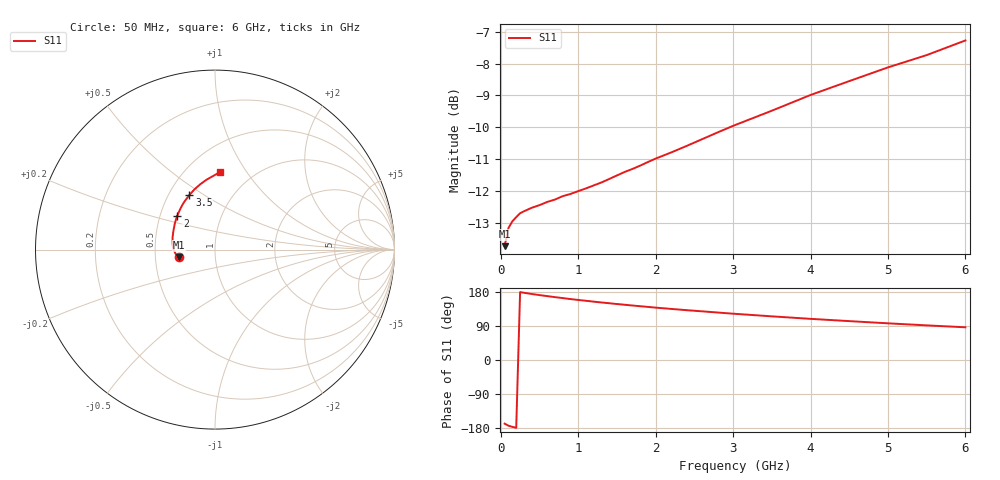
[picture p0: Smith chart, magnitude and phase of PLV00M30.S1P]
! Infineon Technologies  Discrete & RF Semiconductors
! BAR 64-04W /-05W /-06W
! Si PIN Diode in SOT323
! IF = 0.3 mA
! S-Parameters:  October  2008
# GHz  S  MA  R  50
!  f  S11
! GHz  MAG  ANG
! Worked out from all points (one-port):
!   34 points, 50 MHz to 6 GHz, reference 50 ohm
!   lowest |S11| = -13.7 dB at 50 MHz (marker M1), VSWR 1.52, Z = 33.1 - j2.96 ohm
!   |S11| at or under -10 dB: start of sweep to 2.959 GHz
!   S11 on the Smith chart (normalised r, x): 50 MHz: 0.66, -0.06; 2 GHz: 0.61, +0.25; 3.5 GHz: 0.63, +0.43; 6 GHz: 0.72, +0.76
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0.05  0.2057 -168.0
0.1  0.2197 -173.4
0.15  0.225 -176.5
0.2  0.2284 -178.8
0.25  0.2317 179.2
0.3  0.2334 177.4
0.4  0.2363 174.2
0.5  0.2386 171.3
0.6  0.2414 168.6
0.7  0.2434 165.9
0.8  0.2464 163.4
0.9  0.2484 160.8
1.1  0.2535 156.3
1.3  0.2589 151.8
1.6  0.269 145.8
1.8  0.2752 141.9
1.9  0.2788 140.1
2  0.2823 138.2
2.4  0.2955 131.5
2.6  0.3028 128.4
2.8  0.3103 125.3
3  0.3178 122.2
3.5  0.3356 115.2
4  0.3553 108.6
4.5  0.3736 102.6
5  0.3926 96.8
5.5  0.4104 91.4
6  0.4327 86.3
